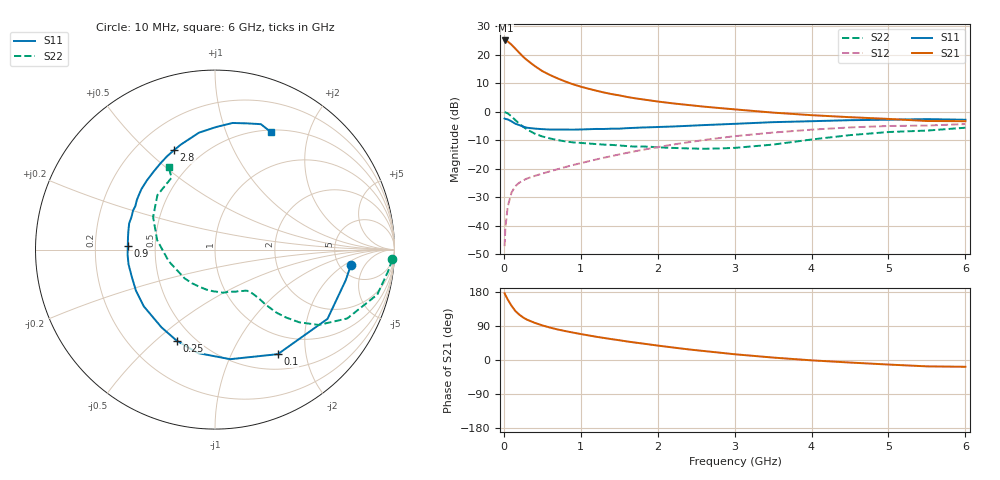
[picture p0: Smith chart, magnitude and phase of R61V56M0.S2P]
! SIEMENS Small Signal Semiconductors
! BFR193
! Si NPN RF Bipolar Junction Transistor in SOT23
! VCE = 1.5 V  IC = 6 mA
! Common Emitter S-Parameters:  May  1996
# GHz  S  MA  R  50
!  f  S11  S21  S12  S22
! GHz  MAG  ANG  MAG  ANG  MAG  ANG  MAG  ANG
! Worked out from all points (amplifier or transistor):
!   36 points, 10 MHz to 6 GHz, reference 50 ohm
!   highest |S21| = 25.0 dB at 20 MHz (marker M1)
!   |S21| within 3 dB of that: start of sweep to 154.2 MHz
!   unconditionally stable (mu >= 1): 838.6 MHz to 2.059 GHz
!   at 250 MHz: K = 0.49, MSG = 21.7 dB, |S12| = -24.1 dB
!   at 1.4 GHz: K = 1.06, MAG = 9.4 dB, |S12| = -15.5 dB
!   at 6 GHz: K = 0.97, MSG = 0.5 dB, |S12| = -4.3 dB
!   S11 on the Smith chart (normalised r, x): 10 MHz: 6.27, -2.61; 100 MHz: 0.71, -1.53; 250 MHz: 0.40, -0.59; 900 MHz: 0.35, +0.02; 2.8 GHz: 0.35, +0.61; 6 GHz: 0.53, +1.45
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0.01  0.7615 -6.6  17.7 176.1  0.0044 87.9  0.988 -3.2
0.02  0.7483 -13.1  17.82 171.5  0.0092 83.6  0.9761 -6.4
0.05  0.7361 -31.6  17.14 159.9  0.0216 74.7  0.9382 -15.5
0.1  0.6796 -59.0  15 143.1  0.0383 63.6  0.8307 -27.5
0.15  0.6164 -82.1  12.79 129.2  0.0497 55.9  0.714 -36.0
0.2  0.5842 -99.4  10.85 119.9  0.057 51.6  0.6198 -40.8
0.25  0.5502 -112.9  9.26 112.4  0.0627 49.2  0.5478 -43.7
0.3  0.5259 -124.5  8.082 106.5  0.0674 48.2  0.4916 -45.7
0.4  0.5073 -141.4  6.37 98.2  0.075 48.1  0.4146 -47.4
0.5  0.4962 -152.8  5.174 91.3  0.0825 49.3  0.3692 -48.0
0.6  0.4875 -162.6  4.413 85.6  0.0904 50.9  0.3407 -48.8
0.7  0.4886 -170.3  3.847 80.5  0.0985 52.5  0.3188 -49.7
0.9  0.4862 177.7  3.034 72.3  0.1167 55.1  0.2905 -52.1
1.1  0.4943 167.3  2.539 64.9  0.1354 56.7  0.2782 -56.0
1.3  0.4993 158.8  2.181 58.2  0.1564 57.4  0.2657 -60.3
1.6  0.516 147.5  1.822 49.0  0.1903 57.6  0.2504 -69.4
2.2  0.552 128.6  1.403 33.0  0.2665 53.8  0.2324 -92.5
2.8  0.5995 112.3  1.164 19.5  0.3461 46.8  0.2273 -124.7
3.5  0.6577 97.8  0.967 6.4  0.4323 35.8  0.266 -165.9
4.5  0.7123 82.1  0.804 -6.7  0.5321 19.9  0.3898 152.2
5.5  0.7441 69.9  0.689 -16.8  0.5733 3.6  0.4681 121.1
6  0.7247 64.4  0.684 -17.9  0.6094 -1.1  0.5254 119.4
